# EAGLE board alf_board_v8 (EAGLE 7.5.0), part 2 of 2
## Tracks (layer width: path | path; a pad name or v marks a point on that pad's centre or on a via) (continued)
DB5  (via drill 0.61) (continued)
  Top 0.254: 73.12,115.5 R7.2 | IC7.19 65.12,68.5 66.62,70 66.62,78.62 68.62,80.62 68.62,112.38 70,113.75 72.75,113.75 73.24,114.24 R7.2 | v67.5,124.88 69.62,122.75 69.62,120.38 73,117 73,115.88 73.12,115.75 73.12,115.62 R7.2 | v183.25,56.88 196.25,56.88 198.5,54.62 IC12.32 | v176,61 v178,61 | v140.5,69 139,70.5 135.12,70.5 132.5,73.12 123.75,73.12 123.75,68.62 122.62,67.5 120.25,67.5 | 120.25,67.5 120.25,65.62 121.88,64 IC2.7 | v117,67.88 120.25,67.88 120.25,67.5
  Bottom 0.254: v67.5,124.88 43.38,124.88 41.75,126.5 CN1.37 | IC2.7 122,64 124.38,66.38 130.75,66.38 IC6.13 | v183.25,56.88 181.75,58.38 181.75,61 v178,61 | v176,61 170.38,66.62 142.88,66.62 v140.5,69 | v117,67.88 111.38,67.88 108.88,65.38 79,65.38 76,68.38 65.12,68.38 IC7.19
DB6  (via drill 0.61)
  Top 0.254: v129.62,47.12 127.75,49 v127.75,59.25 127.75,65.98 IC6.12 | v81.88,121 81.88,115.62 R6.2 82,115.5 82.88,114.62 82.88,101.88 84.25,100.5 84.25,87.62 83.5,86.88 v83.5,74.38 83.5,72.75 v82.5,71.75
  Bottom 0.254: v127.75,59.25 122.38,59.25 122,58.88 IC2.5 | v129.62,47.12 140.25,47.12 143.62,50.5 197.12,50.5 201.12,54.5 IC12.31 | v81.88,121 79.75,123.12 61.12,123.12 60.38,123.88 46.25,123.88 45.5,123.12 42.62,123.12 39.25,126.5 CN1.39 | v82.5,71.75 65.88,71.75 65.12,71 IC7.20 | v83.5,74.38 90.88,74.38 94,71.25 103,71.25 103.88,70.38 104,70.38 104,68.62 105.12,67.5 105.88,67.5 109,69 109,72.62 127.12,72.62 130.75,69 IC6.12
DB7  (via drill 0.61)
  Top 0.254: IC6.11 130.75,71.5 126.88,67.62 126.88,55.73 v126.15,55 | v176,64.25 179.57,60.62 179.57,53.62 187.25,46 187.25,42.38 194.38,42.38 203.7,51.7 IC12.30 | v90.5,114.12 90.5,115.5 R5.2 | 84.38,79.5 84.38,87 84.75,87.38 84.75,100.75 84.38,101.12 v84.38,114 | 84.38,79.5 v84.38,72.62 | CN1.41 36.62,126.5 36.62,121.62 41.05,117.2 v41.05,115.95 | v84.5,79.5 84.38,79.5
  Bottom 0.254: v176,64.25 173.12,67.12 144.88,67.12 139.38,72.62 131.88,72.62 130.88,71.62 IC6.11 130.75,71.62 128.38,74 110.38,74 104.88,79.5 v84.5,79.5 | IC4.13 95.38,110.12 97,111.75 97.75,111.75 97.75,113 96.75,114 90.62,114 v90.5,114.12 84.5,114.12 v84.38,114 84.25,114 83.62,114.62 42.38,114.62 v41.05,115.95 | v84.38,72.62 66,72.62 65.12,73.5 IC7.21 | v126.15,55 124.9,53.75 IC2.3
DR0  (via drill 0.61)
  Top 0.254: v58.5,33.75 58.5,43.25 R22.2 | IC11.3 90.5,10.25 90.5,13.12 89.5,14.12 v89.5,29.1 | v67.75,28.5 68.12,28.12 68.12,11.38 67.25,10.5 52.55,10.5 51,12.05 51,14 50.08,14.92 IC10.2
  Bottom 0.254: v58.5,33.75 65.12,33.75 69.06,29.81 | 69.06,29.81 69.38,29.5 89.1,29.5 v89.5,29.1 | 69.06,29.81 v67.75,28.5
DR1  (via drill 0.61)
  Top 0.254: 53.38,43.12 R21.2 53.46,40.46 53,40 50.3,40 47.45,37.15 47.45,34.95 45.62,33.12 45.62,19.12 47.25,17.5 IC10.3 48.55,16.25 63.75,16.25 65.88,14.12 v65.88,14 | v91.55,13.8 91.55,11.3 91.5,10.25 IC11.4
  Bottom 0.254: v65.88,14 66.62,14.75 90.6,14.75 v91.55,13.8
DR2  (via drill 0.61)
  Top 0.254: 38,21.62 38,31.25 42.3,31.25 42.3,39.05 43.25,40 47,40 48.43,41.43 R20.2 48.38,43.12 | 38,21.62 39.62,20 IC10.15 | v40.62,8.62 38,11.25 38,21.62 | IC11.6 93.59,7.84 v93.25,7.5
  Bottom 0.254: v93.25,7.5 92.5,8.25 41,8.25 v40.62,8.62
DR3  (via drill 0.61)
  Top 0.254: v37.12,17.5 37.12,32.25 41.12,36.25 41.12,40.88 43.38,43.12 R19.2 | IC11.7 94.62,10.12 94.6,8.25 94.6,7.45 v94.85,7.2
  Bottom 0.254: IC10.17 39.62,15 v37.12,17.5 37,17.5 34.12,20.38 27.62,20.38 27.62,19.12 37.25,9.5 42.38,9.5 43.12,8.75 93.5,8.75 v94.85,7.2
DR4  (via drill 0.61)
  Top 0.254: R18.2 107.12,43.25 106.88,43 106.88,36.88 107.62,36.12 107.62,20.75 105.62,18.75 99.12,18.75 IC11.14 99,18.62 95,18.62 v94.38,18
  Bottom 0.254: v94.38,18 74,18 73.5,18.5 60.25,18.5 60.25,16.62 61.88,15 IC9.2
DR5  (via drill 0.61)
  Top 0.254: v102.62,31.38 102.5,31.5 102.5,43.12 102.38,43.25 R17.2 | IC11.16 99,20.75 93,20.75 | v91.12,17.12 93,19 93,20.75 | v93.8,27.2 93,26.4 93,21 93,20.75
  Bottom 0.254: v91.12,17.12 90.75,17.5 62,17.5 IC9.3 | v102.62,31.38 102.38,31.38 98,27 94,27 v93.8,27.2
DR6  (via drill 0.61)
  Top 0.254: 55.44,24.06 55,23.62 52.62,23.62 52.62,21.75 54.25,20.12 IC9.15 | 55.44,24.06 56,24.62 56,29 56.5,29.5 56.5,32.12 58.12,32.12 62.12,36.12 62.12,42 63.38,43.25 R16.2 | v96.38,21.75 99,21.75 IC11.17 | v64,22.62 62.62,24 55.5,24 55.44,24.06
  Bottom 0.254: v64,22.62 93.5,22.62 94.38,21.75 v96.38,21.75
DR7  (via drill 0.61)
  Top 0.254: v97.25,29.88 97.25,43.25 R15.2 | IC11.20 99,24.75 95.28,24.75 | v95.28,28.02 95.28,24.75 | 95.28,24.75 v95.28,23.38 | v64.5,13.88 64.33,13.7 55.59,13.7 IC9.17
  Bottom 0.254: v64.5,13.88 65.88,15.25 91.25,15.25 92.65,16.65 97.65,16.65 98,17 98,23 97.62,23.38 v95.28,23.38 | v95.28,28.02 95.3,28 96,28 97.25,29.25 v97.25,29.88
G  (via drill 0.61)
  Top 0.254: IC11.12 99,16.62 96.72,16.62 96.4,16.3 96.4,12.6 99.12,9.88 122.12,9.88 123.5,11.25 JP3.3 123.5,11.38 123.12,11.75 123.12,28.88 114.38,37.62 v114.38,43.42 | 168.88,114.38 168.62,115.12 R44.2 | v98.5,56.62 96.38,58.75 96.38,91.88 v94.75,93.5
  Top 0.406: v168.88,112.75 168.88,114.38
  Bottom 0.254: v168.88,112.75 163.38,109.25 144.38,109.25 143.75,108.62 128.25,108.62 127.88,109 121.88,109 118.25,105.38 IC21.10 | v98.5,56.62 104.38,56.62 105,56 105,52.8 v114.38,43.42 | v94.75,93.5 95.62,94.38 113.38,94.38 115,96 115,100.15 116.4,101.55 119.95,101.55 120.5,102.1 120.5,104.55 119.7,105.35 IC21.10 | 118.25,105.25 IC21.10
GND  (via drill 0.6, 0.6 pad 0.25, 0.6 pad 2.18, 0.61)  (7 unrouted)
  Top 0.254: 134.38,109.25 134.12,109 C23.2 134,108.88 | 134.38,115.88 C22.- 134.5,116 | 143.5,90.38 R54.1 | 143.5,97.12 R55.1 143.5,97.25 | 144.88,115.25 R48.1 | 140.25,124.38 H5.B3,2 | 143.5,116.5 143.56,116.56 | 135.88,124.38 X2.2 | 134,106.75 133.82,106.62 | 125.88,105.38 IC21.7 | 156.88,90.25 R56.1 | 160.88,90.25 R57.1 160.88,90.38 | 155.88,109.12 R52.1 | 161.88,109.12 R51.1 161.75,109.12 | 161,115.12 R49.1 160.88,115.25 160.5,115.62 | 160.5,124.5 X3.1 | v44.75,23.12 45.12,23.5 45.12,29.5 44.88,29.75 44.88,31.25 44.05,32.08 C4.1 44.12,37 | IC18.8 189.5,19.38 190.25,18.62 190.25,15.62 190.29,15.5 | 19.25,19.88 C2.- | 15.25,20.5 S1.3 15.12,20.62 | 8.62,20.62 S1.4 8.75,20.62 | IC3.7 105.5,69.25 105.88,69.62 105.88,75 106.5,75.62 106.5,81.88 105.62,82.75 IC5.7 105.62,82.88 106.75,84 106.75,85.5 108.38,87.12 108.38,90.75 110.62,93 111,93 | IC16.3 183.25,59 180.75,59 IC16.2 180.75,59.12 180.5,59.38 180.5,64.12 178.25,66.38 IC16.14 | 188.38,66.62 IC16.10 | 204.38,29.75 IC17.13 | 105.62,102.38 IC4.8 | 148.93,15.5 148.88,15.62 147.88,16.62 147.88,29.62 146.25,31.25 IC13.8 | IC18.13 179.25,27.12 178.38,28 178.38,28.62 178,29 178,36.75 178.3,37 | 86.62,10 86.62,10.12 | 109.88,124.38 X1.2@1 | IC11.63 86.62,10.25 86.6,12.47 86.6,22.6 88,24 88,29 88.59,29.59 IC11.32 88.62,32.12 | v51.5,81 51.5,70.5 50.7,69.7 48.9,69.7 48.25,69.05 48.25,64.85 49.75,63.35 IC7.16
  Top 0.406: 228.8,138.95 229,139 | 178.25,72 178.15,71.9 | 178.15,66.58 IC16.14 | R28.1 | 229,72.35 229.35,72 229.15,71.8 229.15,58.85 229.11,58.89 | R66.2 C30.- | C30.- 191.95,113.95 190,113.95 | 190,113.95 C29.2 | IC22.24 190,107.63 190,113.95 | C35.- 211.4,123.05 C34.2 211.3,117.85 R71.1 v213,110 C38.1 | C30.- v192,116 | 229,104.18 229,104 | 229,99.1 229,99 | 214.45,99.8 C37.1 | 229,109.05 229,109 | IC19.10 226.12,23 | 182.46,72 183,72 | 191.46,72 191,72 | 200.46,72 200,72 | 209.46,72 209,72 | C42.2 155,16.05 C43.- 148.93,15.5 X4.1 | C40.2 197,16.05 C41.- 190.29,15.5 X5.1 | 143.5,97.12 143.5,90.38 | 144.88,115.25 143.56,116.56 143.56,120.44 143,121 140.69,121 X2.2 | 125.88,105.38 132.43,105.38 133.82,106.62 | 134,108.88 134,106.75 | 204.38,37 204.38,29.75 | v86.62,3.88 86.62,10 86.62,10.25 | 160.5,124.62 X3.1 | v25.45,74 v25.45,71.12 | 160.88,96.12 160.88,96.25 | 156,107 155.84,107.16 | 143.5,97.25 142.85,97.9 142.85,113.15 144.89,115.19 R48.1 | 204.4,135.15 X7.SH2 | 210.8,134.75 X7.SH1 | 197.65,138.6 arc-90 198,138.95
  Top 0.813: 178.15,71.9 178.15,66.58 | R36.1 159,81.23 | 159,81.23 R28.1 | 229.11,58.89 IC14.7 | IC22.24 190.03,102.5 | 190.03,102.5 IC22.1 | 190.03,102.5 197.65,102.5 IC22.7 197.65,97.3 C36.2 198.3,95.35 198.9,94.75 C27.2 205.25,93.5 C28.- 211.75,93.5 214.45,96.2 v214.45,97.85 214.45,99.8 | IC23.13 229,104.18 | IC23.11 229,99.1 | 226.12,23 229.31,23 | R61.A 182.46,72 | R62.A 191.46,72 | R63.A 200.46,72 | R60.A 209.46,72 | CN1.48 29.16,138.95 29,138.95 | CN1.2 86.66,138.95 87,138.95 | 121.99,77 111,77 111,93 111,102.38 | 111,102.38 111,121 109.88,121 | 109.88,121 105,121 105,138.95 | IC2.10 121.99,77 | 121.99,77 138.4,77 IC6.10 | IC12.1 178.3,37 204.38,37 229.32,37 | 134.38,115.88 134.38,109.25 | 134.5,116 135.88,117.38 135.88,124.38 | 160.88,90.25 159,90.25 | 159,90.25 156.88,90.25 | 160.88,90.38 160.88,96.12 | 159,90.25 159,81.23 | 158.88,107 161.88,107 161.88,109.12 | 158.88,107 156,107 | 161,115.12 161,110.72 161.75,109.12 | 160.5,115.62 160.5,124.5 | 160.88,96.25 158.88,97.25 158.88,107 | 19.25,19.88 15.25,19.88 15.25,20.5 | 8.62,20.62 8.25,21 8.25,26.12 IC1.7 | 8.75,20.62 15.12,20.62 | 188.38,72 188.38,66.62 | 111,102.38 105.62,102.38 | 161,138.95 161,124.62 160.5,124.62 | 109.88,121 109.88,124.38 | 155.84,107.16 R52.1
  Top 1.27: 210.8,134.75 X7.5 204.4,135.15 X7.3 198,134.75 X7.SH3 197.65,138.6
  Top 1.422: 229.35,72 229.32,37 229.31,23 229.3,5 H3.B3,3
  Top 2.184: 9.7,135 9.75,138.95 29,138.95 87,138.95 105,138.95 161,138.95 198,138.95 228.8,138.95 | 229.35,72 209,72 200,72 191,72 188.38,72 183,72 178.25,72 | H1.B3,3 9.7,135 | 229,72.35 229,99 229,104 229,109 229,135 | 229,135 229,139 | H2.B3,3 229,135 | X1.2@1 X1.2@2 X1.2 X2.2@1 X2.2@2 X2.2 142.5,125.39 H5.B3,2 | X6.2 X6.2@2 X6.2@1 167.5,125.46 H6.B3,2 | v9.7,105.55 arc90 9.75,105.6 C47.- 11,111 11,119.39 J1.TIP 9.7,121.91 9.7,135
  Bottom 0.254: 29.62,71.12 IC8.29 29.5,71.12 | 49.75,63.38 IC7.16 | v51.5,81 64.88,81 65,81.12 IC7.24 | IC21.4 125.75,97.75 123.62,99.88 122.12,99.88 C14.1 | 125.75,105.38 IC21.7 | IC9.1 61.88,12.5 59.38,15 58.12,15 58,15.07 | v44.75,23.12 43.75,22.12 43.12,22.12 C13.1 | 40.79,13.12 40.88,13 46.75,13 47.25,12.5 IC10.1 47.38,12.5 | 54.25,12.5 IC9.18 | IC18.13 179.38,27 183.25,23.12 183.25,22.97 | IC17.13 204.5,29.62 208,26.12 208,25.97 | C16.1 134.88,61.88 133.88,61.88 133.88,52.88 132.22,51.22 IC6.19 | IC12.24 219,54.62 220.5,56.12 220.5,62.5 220.62,62.5 C10.1 | C11.1 168.62,38.12 177.12,38.12 178.25,39.25 IC12.1 | 149.99,34.12 150.12,34 151.75,32.38 165.75,32.38 165.84,32.25 | 8,26.38 IC1.7
  Bottom 0.406: C19.1 12,29.1 IC1.7 | IC10.18 40.79,13.12 43,14.66 C13.1 42.25,21.3 37.65,21.3 36.95,22 16,22 15.22,21.22 S1.3 | C20.1 58,15.07 IC9.18 | C12.1 118,68.54 IC2.10 | C16.1 135,69.15 IC6.10 | C18.1 103.24,72.45 IC3.7 | C21.1 103.26,86.1 IC5.7 | C17.1 103.35,105.55 IC4.8 | C14.1 122,104.08 124.52,106.6 | 124.52,106.6 IC21.8 | C9.1 149.99,34.12 IC13.8 | C46.1 183.25,22.97 186.97,22.97 IC18.8 | C45.1 208,25.97 211.66,25.97 IC17.8 | C44.1 225.06,24.06 IC19.10 | C10.1 224.07,62.49 IC14.7 | C5.1 187.4,65.63 IC16.10 | C11.1 168.49,34.17 165.84,32.25 IC20.7 | C15.1 221.45,94.29 IC23.7 | v192,116 191.59,116 X6.2 | IC23.11 C15.1 | C15.1 219.85,97.85 v214.45,97.85 arc-90 213,99.3 v213,110 | 29.62,71.12 32.52,69.72 43.3,69.72 49.75,63.38 | 124.52,106.6 125.75,105.38 | 47.38,12.5 54.25,12.5 | v86.62,3.88 86.62,1 | 1,69.88 16.45,69.9 17.48,71.12 v25.45,71.12 29.5,71.12 | C3.1 v25.45,74 | JP4.2 19.3,11.38 | 1.45,67.65 1.45,66.45 arc-90 1,66
  Bottom 0.813: JP3.2 126,8.73 126,1 | 1,26.38 8,26.38 | 19.3,11.38 19.3,1.79
  Bottom 1.016: 1.45,67.65 1,67.65
  Bottom 2.184: 126,1 86.62,1 19.3,1.79 1,2 1,5 | 1,5 1,26.38 1,66 1,67.65 1,69.88 1,103 arc-90 3.55,105.55 v9.7,105.55 | 1,5 H4.B3,3
  other vias: 176,131 194,135 224,122.3 180,102 176,91 224,112 180,114
  pour Bottom (isolate 0.813): 173,140 230,140 230,109 213,109 213,86 173,86
  pour Top (isolate 1.016): 173,140 230,140 230,109 213,109 213,86 173,86
  pour Bottom (isolate 0.813): 230,0 0,0 0,15 37,15 37,6 230,6
  pour Top (isolate 0.254): 0,140 13,140 13,125 0,125
  pour Top (isolate 0.813): 230,0 207,0 207,3 207,12 230,12
KD0  (via drill 0.61)
  Top 0.254: v207.12,7.75 210.62,11.25 210.62,20.88 209.5,22 IC17.6 | IC11.1 88.62,10.12 88.62,5.7 v93.15,5.7 | v123.88,5.88 127.78,5.88 v127.8,5.85
  Bottom 0.254: v207.12,7.75 129.7,7.75 v127.8,5.85 | v93.15,5.7 123.7,5.7 v123.88,5.88
KD1  (via drill 0.61)
  Top 0.254: v174.62,6.88 175.88,6.88 179,10 179,13 181.38,15.38 v182.88,15.38 | v123.97,3.92 v127.83,3.92 | IC11.2 89.59,7.16 v90.03,6.72
  Bottom 0.254: v182.88,15.38 192.62,15.38 199.25,22 IC17.2 | v90.03,6.72 92.83,3.92 v123.97,3.92 | v127.83,3.92 130.78,6.88 v174.62,6.88
KD2  (via drill 0.61)
  Top 0.254: v138.12,9.5 138.12,4.88 206.25,4.88 213.25,11.88 213.25,31.75 212.75,32.25 v211.62,32.25 | v93.88,15 92.62,15 92.62,10.25 IC11.5
  Bottom 0.254: v211.62,32.25 201.88,32.25 199.38,29.75 IC17.15 | v138.12,9.5 133,14.62 108.5,14.62 108.12,15 v93.88,15
KD3  (via drill 0.61)
  Top 0.254: IC11.8 95.62,10.25 95.62,9.9 v96.83,9.9
  Bottom 0.254: IC17.3 194.25,14.5 148.88,14.5 143,8.62 127.75,8.62 126.5,9.88 96.83,9.88 v96.83,9.9
KD4  (via drill 0.61)
  Top 0.254: IC11.9 99.12,13.62 99,13.5 99,12 99.35,11.65 102.85,11.65 104.5,13.3 v104.5,17.43
  Bottom 0.254: v104.5,17.43 104.5,20.88 105.38,21.75 173.38,21.75 173.57,22.15 176.57,22.15 176.75,21.88 186.62,21.88 188,20.5 arc-45 188.25,19.9 188.25,17.95 188.9,17.3 189.9,17.3 191.1,18.5 193.25,18.5 196.75,22 IC17.1
KD6  (via drill 0.61)
  Top 0.254: v138.12,19.5 144.75,12.88 144.75,5.38 206,5.38 212,11.38 IC17.7 | v105.38,20.5 102.25,23.62 99.12,23.62 IC11.19
  Bottom 0.254: v138.12,19.5 137.62,20 105.88,20 v105.38,20.5
KJ0  (via drill 0.61)
  Top 0.254: v134.88,29.62 v134.88,43.5
  Bottom 0.254: v134.88,43.5 133.88,44.5 126.75,44.5 126.75,46.38 122,51.12 IC2.2 | v134.88,29.62 135.12,29.88 163.38,29.88 163.5,30 171.38,30 174.25,27.12 IC18.15
KJ1  (via drill 0.61)
  Top 0.254: v123.75,46.12 123.75,54.5 122,56.25 IC2.4 | v169.25,28.12 169.25,21.88 171.62,19.5 IC18.1 | v134,28.75 134,43.12 v133.5,43.62
  Bottom 0.254: v123.75,46.12 126.25,43.62 v133.5,43.62 | v134,28.75 137.38,28.75 138,29.38 163.62,29.38 163.75,29.5 167.88,29.5 v169.25,28.12
KJ2  (via drill 0.61)
  Top 0.254: v120.25,46.12 120.25,59.62 121.88,61.25 IC2.6 | v120.25,42.38 124.12,38.5 124.12,32.62 v135.88,20.88
  Bottom 0.254: v120.25,42.38 v120.25,46.12 | v135.88,20.88 136.12,21.12 172.62,21.12 174.25,19.5 IC18.2
KJ3  (via drill 0.61)
  Top 0.254: v124.62,47.25 124.62,63.75 122,66.38 IC2.8 | v135.88,19.12 123.62,31.38 123.62,36.12 118.75,41 118.75,43.25 119.38,43.88 v121.12,43.88
  Bottom 0.254: v124.62,47.25 124.38,47 123.38,47 121.12,44.75 v121.12,43.88 | v135.88,19.12 137.25,17.75 175.12,17.75 176.75,19.38 IC18.3
KJ4  (via drill 0.61)
  Top 0.254: v118,75.88 118,75.25 114.38,71.62 IC2.11 | v146.88,68.88 147.75,68 v147.75,65.5 | v152.5,60.75 157.62,55.62 157.62,25.77 160.4,23 164.2,23 165.1,23.9 167.8,23.9 168.25,23.45 168.25,20.75 v172.62,16.38
  Bottom 0.254: v118,75.88 118.38,76.25 139.5,76.25 v146.88,68.88 | v152.5,60.75 v147.75,65.5 | v172.62,16.38 173,16.75 181.75,16.75 184.38,19.38 IC18.6
KJ5  (via drill 0.6 pad 0.41)
  Top 0.406: v217,89 v217,86 | v209,88 v200,88 | v112.2,75.45 111.3,74.55 v111.3,71.75 | v112,69 111.75,68.75 v111.75,66.4
  Bottom 0.406: IC23.8 225.26,89 v217,89 | v217,86 214,86 212,88 v209,88 | v112.2,75.45 112.2,78.2 119,85 133,85 136,88 v200,88 | v111.3,71.75 112,71.05 v112,69 | v111.75,66.4 111.8,66.45 IC2.13
KJ6  (via drill 0.61)
  Top 0.254: IC2.15 112.62,59.62 112.62,36.62 122.25,27 v122.25,19.12
  Bottom 0.254: v122.25,19.12 124.12,17.25 177.12,17.25 179.25,19.38 IC18.4
KJ7  (via drill 0.61)
  Top 0.254: v110.88,59.75 110.88,70.12 v116.62,75.88 | v214.75,81.38 215,81.62 215,92 217.02,94.02 IC23.6
  Bottom 0.254: v110.88,59.75 114.25,56.38 IC2.17 | v116.62,75.88 118.12,77.38 181.12,77.38 182,76.5 209.88,76.5 v214.75,81.38
N$1
  Top 0.406: R65.1 199.1,92 212,92 215.55,95.55 215.55,97.7 216.95,99.1 IC23.4
N$2
  Bottom 0.254: C1.1 28.12,37.62 29.5,39 29.5,41.88 28.12,41.88 R1.2 | IC1.2 8.12,39 5.88,40.65 5.88,42.9 6.97,44 19,44 21.1,41.9 R1.2 | 28,42 R1.2
N$3  (via drill 0.61)
  Top 0.254: v13.62,36.38 8.25,36.38 IC1.3
  Bottom 0.254: v13.62,36.38 14.62,35.38 18.38,35.38 20,37 22,37 23.37,35.63 C1.2 | 27.75,36 28,35.75 C1.2 | C1.2 29.63,35.63 30,36 30,37 30.53,37.53 R2.1
N$4
  Bottom 0.254: R1.1 28,40 27.75,39.75 21.12,39.75 Q1.1 21,39.75 18.25,42.5 9.25,42.5 8.25,41.5 IC1.1
N$5  (via drill 0.6, 0.61)
  Top 0.254: v177.12,36.38 177.12,29.12 177.88,28.38 177.88,26.38 178.38,25.88 178.38,23 181.88,19.5 IC18.5 | v190,43.25 199.62,52.88 199.62,55.75 192.62,62.75 v181.38,62.75 | v178.12,64.5 176.5,66.12 176.5,74.5 177.1,75.1 v177.3,75.1 | v207.75,75.1 207.75,84.75 211,88 211,90 217.56,96.56 IC23.5
  Bottom 0.254: v181.38,62.75 179.62,64.5 v178.12,64.5 | v177.12,36.38 188.38,36.38 189.7,37.7 189.7,42.95 v190,43.25 | v207.75,75.1 v177.3,75.1
N$6  (via drill 0.61)
  Top 0.254: v175.55,21.12 170.75,21.12 170.75,25.25 v170.12,25.88 | v164.12,28.62 163.12,29.62 163.12,49 165.12,51 165.12,64.75 v170.25,69.88
  Top 0.406: v214.5,76 220,76 222,78 222,93 223.02,94.02 IC23.9
  Bottom 0.254: v175.55,21.12 185.25,21.12 186.88,19.5 IC18.7 | v170.12,25.88 167.38,28.62 v164.12,28.62 | v170.25,69.88 176.38,76 v214.5,76
N$7  (via drill 0.61)
  Top 0.254: v102.5,55.25 104.5,57.25 104.5,75.75 105.5,76.75 IC3.8 | v20.82,52.15 20.82,44.83 18,42 18,40 16.94,38.94 IC1.13
  Bottom 0.254: v102.5,55.25 99.38,52.12 20.85,52.12 v20.82,52.15
N$8
  Top 0.254: 22.62,16.88 R3.1 | 19.38,16.88 C2.+ 19.25,16.75 | 15.25,16.12 S1.1 15.12,16.12 | 8.12,31.25 IC1.5 | 8.62,16.12 S1.2 8.75,16.12
  Top 0.406: JP4.1
  Top 0.813: 19.38,16.88 22.62,16.88 | 19.25,16.75 15.25,16.75 15.25,16.12 | 8.12,31.25 4.38,29.5 4.38,18.38 8.62,16.12 | 8.75,16.12 15.12,16.12 | JP4.1 C2.+
N$9
  Bottom 0.254: IC4.7 102.88,102.38 98.25,97.75 81.25,97.75 JP1.1
N$10  (via drill 0.61)
  Top 0.254: v101.25,55.75 101.5,56 101.5,75.75 100.5,76.75 IC3.10 | v35.4,38.75 35.4,41.4 36.35,42.35 v36.35,53
  Bottom 0.254: v36.35,53 98.5,53 v101.25,55.75 | IC1.10 15.88,31.25 16.75,30.38 33.38,30.38 34.65,31.65 34.65,38 v35.4,38.75 | IC3.12 95.38,76.75 97,75.12 98.75,75.12 100.38,76.75 IC3.10
N$11  (via drill 0.61)
  Top 0.254: v96.88,107 96.88,70.25 97.88,69.25 IC3.4
  Bottom 0.254: v96.88,107 95.62,108.25 94.62,108.25 92.88,110 IC4.14
N$12  (via drill 0.61)
  Top 0.254: v108.5,73.62 109,73.12 109,57 v108.62,56.62
  Bottom 0.254: IC2.1 121.88,48.62 120.88,47.62 112.62,47.62 112.62,49.5 114.25,51.12 IC2.19 114.12,51.12 v108.62,56.62 | v108.5,73.62 104.5,73.62 104.5,77.38 103.38,78.5 99.62,78.5 98,76.88 IC3.11
N$13
  Top 0.254: IC3.1 90.25,69.25 89.25,70.25 89.25,109 90.25,110 IC4.15
N$14
  Top 0.254: IC19.11 226,25.62 221,30.62 218.5,30.62 IC19.2 | IC18.12 182,27.12 183.62,28.75 185.88,28.75 185.88,24.62 188.25,22.25 188.25,13.25 190,11.5 199.88,11.5 199.88,10.38 X5.12
  Bottom 0.254: IC17.12 207,29.75 208.62,31.38 217.75,31.38 218.38,30.75 IC19.2 | 198.81,9.19 199.88,10.25 X5.12 | 198.81,9.19 198.25,8.62 160.25,8.62 158.62,10.25 X4.12 | IC19.11 226.12,25.5 227.75,23.88 227.75,14.5 213.88,14.5 208.5,9.12 198.88,9.12 198.81,9.19
N$15  (via drill 0.61)
  Top 0.254: v83.75,42.38 83.75,61.88 83.88,62 R25.2 | IC11.21 99,25.75 97.12,25.75 96.38,26.5 v96.38,40.75
  Bottom 0.254: v83.75,42.38 85.38,40.75 v96.38,40.75
N$16
  Top 0.254: 208.75,54.62 IC12.28
  Top 0.813: R38.2 204.75,60.5 208.75,56.25 208.75,54.62
  Bottom 0.254: IC12.25 216.38,54.62 214.75,56.25 210.5,56.25 208.88,54.62 IC12.28
N$17  (via drill 0.61)  (1 unrouted)
  Top 0.254: 146.88,115.25 R48.2 146.88,115.12 | 146.88,109.25 R43.1 146.88,109.12
  Top 0.406: 146.88,115.25 146.88,119.62 D1.A | 146.88,115.12 146.88,109.25 | v147.38,107 146.88,107.5 146.88,109.12
  Bottom 0.406: 168.62,103.25 167.47,104.4 156.72,104.4 154.28,106.85 147.53,106.85 v147.38,107
N$18
  Top 0.254: 139.25,115.88 139.88,115.25 R47.2 | 139.25,119.62 D1.C
  Top 0.406: 139.25,119.62 139.25,115.88
N$19  (via drill 0.61)
  Top 0.254: 162.75,115.25 R49.2
  Top 0.406: 162.75,115.25 162.72,115.28 v162.72,120.95 | v171.5,81 171,81.5 171,105 170.38,105.62 168.75,105.62 168.69,105.69 T1.E
  Bottom 0.254: R61.E 185,81 v171.5,81
  Bottom 0.406: X3.2 157.77,124.23 161.05,120.95 v162.72,120.95 163.1,120.95 163.6,120.45 170.6,120.45 170.6,106.3 169.99,105.69 T1.E
N$20  (via drill 0.6 pad 0.25)
  other vias: 195.1,112.45
N$21  (via drill 0.61)
  Top 0.254: 166.38,115.62 166.75,115.25 R44.1 | 163.75,109.25 R51.2
  Top 0.406: v166.38,116.75 166.38,115.62 | v163.75,113.12 163.75,109.25 | T2.B 161.75,103 164,103 165,104 165,109 164.76,109.24 R51.2
  Bottom 0.406: v166.38,116.75 165.38,115.75 163.75,115.75 | 163.75,115.75 152.65,115.75 D2.A | 163.75,115.75 v163.75,113.12
N$22  (via drill 0.61)
  Top 0.254: 140,109.12 R50.2
  Top 0.406: 140,109.12 140.5,108.62 v140.5,107.62
  Bottom 0.254: v140.5,107.62 140.88,108 152.52,108 D2.C
N$23  (via drill 0.61)
  Top 0.254: 157.62,109.25 R52.2 157.75,109.12 | 155,124.5 X3.3
  Top 0.406: 157.62,109.25 157.62,121.85 156.88,122.62 155,124.5 | v159.9,108.28 158.94,109.24 R52.2 | v169.38,107.12 170.88,107.12 172,106 172,83 173,82 196.54,82 R62.E
  Bottom 0.406: v169.38,107.12 169.1,107.4 161.65,107.4 161.63,107.38 | 161.63,107.38 T2.E | v159.9,108.28 160.79,107.38 161.63,107.38
N$24  (via drill 0.6 pad 0.25)
  Top 0.406: IC22.17 198.92,105.45 v198.9,105.45 | v188.15,105.1 186.05,105.1 arc90 R67.2
  Bottom 0.406: v198.9,105.45 arc-90 198.55,105.1 v188.15,105.1
N$25
  Top 0.254: IC12.27 211.38,54.62 212.88,56.12 212.88,67.5 213.62,68.25 219,68.25 219,66.62 IC14.11
N$26  (via drill 0.61)
  Top 0.254: IC5.4 98,82.75 99.38,81.38 99.38,56.38 102.62,53.12 102.62,46.17 103.8,45 103.8,41.3 104.75,40.35 104.75,37.45 106.08,36.12 v106.08,35.88 | v171.75,25 172.75,26 172.75,27.62 176,30.88 176,39.12 177.5,40.62 177.5,43.62 186.25,43.62 186.75,43.12 186.75,41 210,41 222.62,53.62 222.62,65 IC14.9 | v147,26.38 144,29.38 144,33 144.88,33.88 146.12,33.88 IC13.7
  Bottom 0.254: v106.08,35.88 144.25,35.88 146.12,34 IC13.7 | v171.75,25 150.5,25 149.12,26.38 v147,26.38
N$27  (via drill 0.61)
  Top 0.254: v210.12,48.75 215,53.62 215,65.5 214,66.5 IC14.13 | v166.75,37.83 166.75,37.88 v169.88,41
  Bottom 0.254: v169.88,41 170.25,40.62 174.62,40.62 176.25,42.25 185.12,42.25 185.5,41.88 187.38,41.88 194.25,48.75 v210.12,48.75 | v166.75,37.83 162.95,37.83 161.57,36.45 IC13.11
N$28  (via drill 0.61)
  Top 0.254: v103,87.12 103,85.38 100.5,82.88 IC5.5 | v150,60.75 152.12,58.62 152.12,35.62 153.75,34 IC13.10
  Top 0.406: v144,65 143,66 143,80 135.12,87.88 v130.25,87.88
  Bottom 0.254: v144,65 148.25,60.75 v150,60.75
  Bottom 0.406: v130.25,87.88 110.88,87.88 110,87 108,87 107,88 104.85,88 104.1,87.25 103.12,87.25 v103,87.12
N$29  (via drill 0.61)
  Top 0.254: v205.88,41.88 217.62,53.62 217.62,62.75 | 217.62,62.75 217.62,65.5 216.62,66.5 IC14.12 | IC14.10 221.5,66.5 217.75,62.75 217.62,62.75
  Bottom 0.254: v205.88,41.88 192.5,41.88 192.5,38.75 189.25,35.5 171.75,35.5 166.75,30.5 154.62,30.5 153.88,31.25 IC13.9
N$30  (via drill 0.61)
  Top 0.254: IC18.10 187,27.12 187,28 191,32 R41.1 191.12,32.12 194.38,35.38 v198,35.38 | v206.38,35.38 212,29.75 IC17.10
  Bottom 0.254: v198,35.38 v206.38,35.38
N$31
  Top 0.254: IC12.29 206.25,54.5 207.88,52.88 210.05,52.88 210.05,68.75 226.62,68.75 226.62,66.62 IC14.8
N$32
  Top 0.406: 154,74.86 R33.2 R34.1 150.64,70.81 R37.1 150.56,70.81 R35.1 | 154,74.86 150.41,74.86 C8.+ | R36.2 154,80.22 154,74.86
N$33
  Top 0.406: 164,74.86 R31.2 R32.1 167.31,70.81 R29.1 R30.1 | 164,74.86 167.54,74.86 C7.+ | R28.2 164,80.16 164,74.86
N$34  (via drill 0.6)
  Top 0.254: 138.12,103.12 R45.1 | 139.38,90.38 D3.A
  Top 0.406: R54.2 145,89.95 145,88 140,88 139.43,88.57 D3.A 138.74,90.26 137,92 137,102 138.12,103.12 138.12,100 v141,100
  Bottom 0.406: v141,100 144.16,103.16 T3.B
N$35  (via drill 0.61)
  Top 0.254: 186.19,14.56 190.38,10.38 191.62,10.38 X5.9 | 186.19,14.56 185.88,14.88 185.88,21.12 185.38,21.62 185.38,26.12 184.5,27 IC18.11 | v175.12,34.62 175.12,39 172.5,41.62 IC20.12 | X4.9 150.38,10.25 154.62,6 186.12,6 186.12,14.5 186.19,14.56 | IC17.11 208.12,28.38 v208.12,19.75
  Bottom 0.254: IC17.11 209.5,29.62 211.12,28 216.25,28 217.88,29.62 222.5,29.62 226,33.12 IC19.14 | v175.12,34.62 181,28.75 182.75,28.75 184.38,27.12 IC18.11 | X5.9 191.75,10.38 192.88,11.5 202.38,11.5 202.65,11.78 202.65,14.28 v208.12,19.75
N$36  (via drill 0.6)
  Top 0.254: v161,34 160,33 160,26 160.95,25.05 R39.1 162,25 166,25 C39.1
  Bottom 0.254: IC20.5 163.6,36.6 v161,34
N$37  (via drill 0.6, 0.61)
  Top 0.254: v176.88,52.38 177.05,53.1 177.05,58.35 178.12,58.88 IC16.1 | v161.9,39.15 161.9,36.86 R26.2 | Q2.2 171.25,57 168.25,57 168.25,41.25 166.14,39.14 IC20.4
  Bottom 0.254: v176.88,52.38 171.38,52.38 Q2.2 | IC20.4 v161.9,39.15
N$38  (via drill 0.61)
  Top 0.254: v161.5,48.12 161.5,48.38 160,48.38 R27.1 | Q2.1 166.38,52.38 165.62,51.62 165.62,47.62 164.88,46.88 IC20.1
  Bottom 0.254: v161.5,48.12 162.75,46.88 164.75,46.88 IC20.1
N$39  (via drill 0.6)
  Top 0.254: C6.1 159.99,45 | 159.99,45 159.99,46.56 R27.2 | v162,45 159.99,45
  Bottom 0.254: IC20.2 162.78,44.22 v162,45
N$40  (via drill 0.6)
  Top 0.254: v161.95,41.7 arc0 C6.2 159.99,38.76 R26.1
  Bottom 0.254: IC20.3 v161.95,41.7
N$41  (via drill 0.6)
  Top 0.406: R53.2 134.71,96.71 v135,97
  Bottom 0.406: v135,97 135.88,97.88 D3.C
N$42  (via drill 0.61)
  Top 0.254: 145.38,97.25 R55.2 145.38,97.12 | 145.38,100.5 T3.E
  Top 0.406: 145.38,100.5 145.38,97.25 | v149.25,86.12 149.25,93.33 R55.2 | v150.38,103.88 150.38,122.72 X3.4
  Bottom 0.254: R63.E 202.12,81.88 179.5,81.88 177.38,84 166,84 163.88,86.12 v149.25,86.12 | T3.E
  Bottom 0.406: v150.38,103.88 146.12,100.62 T3.E
N$43  (via drill 0.6, 0.61)
  Top 0.254: 162.75,90.25 R57.2 | X3.5 149.5,124.5 149.5,102.5 151.4,100.6 T4.E
  Top 0.406: 162.75,90.25 v162.75,92.75 163,93 169,93 169.45,92.55 169.45,80 179,80 180,79 v180,74
  Bottom 0.254: 152.38,100.5 T4.E
  Bottom 0.406: v162.75,92.75 153,100.5 152.38,100.5 | R60.E 217,76 217,74 v180,74
N$44  (via drill 0.61)
  Top 0.254: 132.12,109 C23.1 132.25,108.88 132.05,108.38 | 128.88,112.25 L1.2 128.88,112.38 | 131.38,115.88 C22.+
  Top 0.406: v132.05,107.2 132.05,108.38
  Top 0.813: 131.38,115.88 128.88,113.38 128.88,112.38 | 128.88,112.25 128.88,111.12 131.06,108.94 C23.1
  Bottom 0.254: 161.75,100.62 T2.C 161.62,100.62 | 168.62,100.62 T1.C | 145.38,105.75 T3.C 145.25,105.75 | 152.25,105.75 T4.C 152.38,105.62
  Bottom 0.406: 168.62,100.62 161.75,100.62 | 152.25,105.75 145.38,105.75 | v132.05,107.2 134.75,105.75 145.25,105.75 | 152.38,105.62 153.38,105.62 158.42,100.58 T2.C
N$45  (via drill 0.6)
  Top 0.406: X3.9 148.58,127.42 v144,132
  Bottom 0.813: R58.1 142.41,132 v144,132
N$46
  Top 0.254: R40.2 201,34 201.75,33.25 201.75,29.75 IC17.14 201.84,27.56 205.65,23.75 205.65,20.15 207.1,18.7 209.49,18.7 X5.8
N$47
  Top 0.254: IC19.9 226,20.62 218.5,28.12 IC19.3
N$48  (via drill 0.61)
  Top 0.254: v179,29.25 179,34 R42.1 | X4.8 168.25,12.88 172.38,12.88 177.88,18.38 177.88,25.62 176.88,26.62 176.88,27 IC18.14
  Bottom 0.254: v179,29.25 176.88,27.12 IC18.14
N$49
  Top 0.254: IC19.12 226,28.25 224.12,28.25 219.25,33.12 218.5,33.12 IC19.1
N$50
  Top 0.254: IC20.11 172.5,39.12 174.12,37.5 174.12,33.25 172.5,31.62 IC20.8 172.38,31.5 169.5,31.5 167.9,29.9 C39.2
N$51
  Top 0.254: 170.75,36.5 172.38,36.5 IC20.10 | 170.75,36.5 168.12,36.5 166.5,34.88 166.5,29.5 163.95,26.95 R39.2 | 170.75,36.5 170.75,42.5 172.38,44.12 IC20.13
N$52
  Top 0.406: C26.1 R61.S
N$53  (via drill 0.61)
  Top 0.254: v167.38,34.5 172.38,34.5 172.38,34.12 IC20.9
  Bottom 0.254: v167.38,34.5 165.25,34.5 164.88,34.12 IC20.6
N$54
  Top 0.406: C25.1 R62.S
N$55
  Top 0.406: C24.1 193.85,92.15 202.46,83.54 R63.S
N$56
  Top 0.406: IC22.3 192.57,98.57 191.65,97.65 C25.2
N$57
  Top 0.406: IC22.2 191.3,99.1 C26.2
N$58
  Top 0.406: IC22.4 C24.2
N$59
  Top 0.406: 214.88,106.72 arc-90 C38.2
  Top 0.813: IC23.1 214.88,106.72 | C38.2 210.44,107.15 arc90 Q3.1
  Bottom 0.406: R64.2 IC23.1
N$60
  Top 0.406: 217.64,101.75 IC23.3
  Top 0.813: 217.64,101.75 C37.2 210.84,101.75 arc-90 Q3.2 | IC23.3 IC23.2
  Bottom 0.406: R64.1 IC23.2
N$61  (via drill 0.6 pad 0.41)
  Top 0.406: IC22.10 201.46,98.54 202.1,97.9 v202.1,96.4
  Bottom 0.406: v202.1,96.4 202.1,93.44 R60.S
N$62  (via drill 0.6, 0.61)
  Top 0.254: 138,109.25 R50.1 137.88,109.12 | 138,115.12 R47.1 | 134.62,92.5 R53.1 | v109.25,88.75 109.25,74.88 109.88,74.25 109.88,73.62 109.5,73.25 109.5,52.62 109.12,52.25 109.12,18.12 115.88,11.38 JP3.9
  Top 0.406: 138,115.12 138,109.25 | 134.62,92.5 131.5,92.5 130,94 | 130,94 130,99 | 130,99 128.73,100.27 IC21.5 | 137.88,109.12 136,107.25 136,105 130,99 | v129,90 130,91 130,94
  Bottom 0.406: v129,90 127.75,88.75 v109.25,88.75
N$63
  Top 0.406: IC22.6 196.38,92.8 R65.2
N$64  (via drill 0.6 pad 0.25)
  Top 0.406: IC22.20 v195.11,112.44 v195.1,112.45 | v195.1,115.45 195.15,115.45 R68.2
  Bottom 0.406: v195.1,112.45 v195.1,115.45
N$65
  Top 0.406: IC22.9 C36.1
N$66
  Top 0.406: IC22.18 R66.1
N$67
  Top 0.406: IC22.16 R69.2
N$68
  Top 0.406: IC22.15 201.46,112.46 R70.2
N$69
  Top 0.813: R68.1 C33.+
N$70
  Top 0.406: 204.7,122.7 C32.+
  Top 0.813: R69.1 202.6,120.6 204.7,122.7
N$71  (via drill 0.6 pad 0.25)
  Top 0.406: R70.1 v204.75,115.9 | v214.9,115.9 218,115.9 C31.+
  Bottom 0.406: v204.75,115.9 v214.9,115.9
N$72
  Top 0.406: IC22.14 202.73,110.73 207,115 207,121.4 C35.+
N$73
  Top 0.406: C34.1 209.5,114.15 R71.2 209.35,114 209,114 204,109 IC22.13
N$74  (via drill 0.6 pad 0.25)
  other vias: 195.1,115.45
N$75
  Top 0.813: C33.- X6.1
N$76  (via drill 0.61)
  Top 0.254: v36,20.38 36,36 R24.1 | v42.38,12 v44.25,13.88
  Bottom 0.254: v36,20.38 38.88,17.5 39.62,17.5 IC10.16 39.75,17.38 41.38,17.38 41.38,14.5 40.75,13.88 38,13.88 38,12 38.62,11.38 41.75,11.38 v42.38,12 | v44.25,13.88 50.75,13.88 54.25,17.38 IC9.16
N$77  (via drill 0.61)
  Top 0.254: 49,35 50,36 R23.1 | 49,24.25 49,35 | 49,24.25 47.38,22.62 IC10.5 | v46.12,35.5 46.12,36.88 46,37 C4.2 | v48.62,35.25 48.88,35 49,35 | 49,24.25 49,19 58.62,19 61.96,22.34 IC9.5
  Bottom 0.254: v46.12,35.5 46.38,35.25 v48.62,35.25
N$78
  Top 0.813: C32.- 201,126.85 X7.6
N$79
  Top 0.813: C31.- 210.9,129.25 X7.8
N$80  (via drill 0.6 pad 0.25)
  other vias: 192.05,109.5
N$81  (via drill 0.6 pad 0.25)
  other vias: 187.45,109.4
N$82  (via drill 0.6 pad 0.25)
  other vias: 196.4,109.5
N$83  (via drill 0.6 pad 0.25)
  other vias: 192,116
N$84  (via drill 0.6 pad 0.25)
  other vias: 204.75,115.9
N$85  (via drill 0.6 pad 0.25)
  other vias: 214.9,115.85
N$86  (via drill 0.6 pad 0.25)
  other vias: 198.95,105.45
N$87  (via drill 0.6 pad 0.25)
  other vias: 188.1,105.1
N$88  (via drill 0.6)
  other vias: 213,110
N$89  (via drill 0.6)
  other vias: 212.15,96.35
N$90  (via drill 0.6)
  other vias: 202.1,96.4
N$91  (via drill 0.6 pad 2.18)
  other vias: 9.7,105.55
N$93  (via drill 1 pad 1.78)
  other vias: 9.41,99.06
N$94  (via drill 1 pad 1.78)
  other vias: 9.41,96.52
N$95  (via drill 1 pad 1.78)
  other vias: 9.41,93.98
N$96  (via drill 1 pad 1.78)
  other vias: 9.41,91.44
N$97  (via drill 1 pad 1.78)
  other vias: 9.41,88.9
N$98  (via drill 1 pad 1.78)
  other vias: 9.41,86.36
N$99  (via drill 1 pad 1.78)
  other vias: 9.41,83.82
N$100  (via drill 1 pad 1.78)
  other vias: 9.41,81.28
N$101  (via drill 1 pad 1.78)
  other vias: 9.41,78.74
N$102  (via drill 1 pad 1.78)
  other vias: 9.41,76.2
N$103  (via drill 1 pad 1.78)
  other vias: 6.87,76.2
N$104  (via drill 1 pad 1.78)
  other vias: 6.87,78.74
N$105  (via drill 1 pad 1.78)
  other vias: 6.87,81.28
N$106  (via drill 1 pad 1.78)
  other vias: 6.87,83.82
N$107  (via drill 1 pad 1.78)
  other vias: 6.87,86.36
N$108  (via drill 1 pad 1.78)
  other vias: 6.87,88.9
N$109  (via drill 1 pad 1.78)
  other vias: 6.87,91.44
N$110  (via drill 1 pad 1.78)
  other vias: 6.87,93.98
N$111  (via drill 1 pad 1.78)
  other vias: 6.87,96.52
N$112  (via drill 1 pad 1.78)
  other vias: 6.87,99.06
N$113  (via drill 1 pad 1.78)
  other vias: 4.33,99.06
N$114  (via drill 1 pad 1.78)
  other vias: 4.33,96.52
N$115  (via drill 1 pad 1.78)
  other vias: 4.33,93.98
N$116  (via drill 1 pad 1.78)
  other vias: 4.33,91.44
N$117  (via drill 1 pad 1.78)
  other vias: 4.33,88.9
N$118  (via drill 1 pad 1.78)
  other vias: 4.33,86.36
N$119  (via drill 1 pad 1.78)
  other vias: 4.33,83.82
N$120  (via drill 1 pad 1.78)
  other vias: 4.33,81.28
N$121  (via drill 1 pad 1.78)
  other vias: 4.33,78.74
N$122  (via drill 1 pad 1.78)
  other vias: 4.33,76.2
N$123  (via drill 1 pad 1.78)
  other vias: 9.51,71.7
N$124  (via drill 1 pad 1.78)
  other vias: 6.97,71.7
N$125  (via drill 1 pad 1.78)
  other vias: 4.43,71.7
N$126
  Top 0.406: T4.B 153.86,103.14 156.76,100.24 R46.1 156.76,93.76 155,92 155,90.3 R56.2
PBANK  (via drill 0.61)
  Top 0.254: v73.38,119.25 71.5,121.12 v71.5,122.25 71.5,126.42 CN1.13 | v58.48,122.17 58.48,117.03 57.45,116 57.45,113.2 56.5,112.25 56.5,65.88 56.88,65.5 56.88,59.75 55.5,58.38 v55.5,57.38 | v21.25,55.38 21.25,54.38 13,46.12 13,39 15.6,36.4 IC1.12
  Bottom 0.254: v21.25,55.38 23.07,57.2 55.33,57.2 v55.5,57.38 | v71.5,122.25 58.55,122.25 v58.48,122.17 | v73.38,119.25 95.12,119.25 95.5,118.88 105.5,118.88 105.5,110.12 IC4.9
R  (via drill 0.61)
  Top 0.254: v144.38,110.75 144.38,109.75 144.88,109.25 R43.2 | v109.88,96.75 106.62,93.5 106.62,86.12 104,83.5 104,74.12 v103.62,73.75 | v106.75,70.62 107.12,70.25 107.12,45.38 108.25,44.25 108.25,40.25 107.38,39.38 107.38,37.12 108.12,36.38 108.12,14.5 v107.75,14.12 | v103.2,14.12 102.88,14.12 101.26,15.74 IC11.11
  Bottom 0.254: v144.38,110.75 144,110.38 116.25,110.38 116.25,102.75 | IC21.11 118.12,102.88 116.38,102.88 116.25,102.75 | JP3.1 126,11.38 123.25,14.12 v107.75,14.12 v103.2,14.12 | 116.25,102.75 110.25,96.75 v109.88,96.75 | v106.75,70.62 v103.62,73.75
RES  (via drill 0.61)  (1 unrouted)
  Top 0.254: 8.25,28.88 IC1.6 | 15.75,28.88 IC1.9 | v26.12,29.5 27,30.38 27,69.9 31.3,69.9 32.25,70.85 32.25,79 31.15,80.1 27.9,80.1 26.55,81.45 26.55,101.15 27.8,102.4 28.8,102.4 30.25,103.85 30.25,125.12 31.62,126.5
  Top 0.813: 15.75,28.88 8.25,28.88
  Bottom 0.254: IC1.9 15.88,28.88 25.5,28.88 v26.12,29.5
SL  (via drill 0.6)
  Top 0.254: 150.12,78.12 C8.-
  Top 0.406: v148.05,130.8 156.38,130.8 X3.7 156.38,127.38 155,126 148,126 148,122 148.6,121.4 148.6,99.4 151,97 151,79 150.12,78.12
  Bottom 0.406: v148.05,130.8 133.8,130.8 132,129 118,129 X1.1
SOUND-IN  (via drill 0.61)
  Top 0.254: v49,112.88 49,124.25 46.75,126.5 CN1.33 | v90.12,105 91.75,103.38 91.75,97.75 v96,93.5 | 151.78,67.78 v152,68
  Top 0.406: R37.2 151.78,67.78 153.3,66.25 165,66.25 167.35,68.6 R29.2 | v139.62,73.62 140,74 140,79 133,86 124,86 122,88 122,92 120.25,93.75 v120,93.75
  Bottom 0.254: v49,112.88 55.75,106.12 89,106.12 v90.12,105 | v96,93.5 96.25,93.75 v120,93.75 | v139.62,73.62 145.25,68 v152,68
SR  (via drill 0.6, 0.61)  (1 unrouted)
  Top 0.254: 167.88,78.25 C7.-
  Top 0.406: v159.15,129.7 X3.6 | 167.88,78.25 167.82,78.3 v167.82,91.55
  Bottom 0.406: v167.82,91.55 171.6,97.88 171.6,121.62 164.12,121.62 162.4,123.35 162.4,127.4 162.38,127.42 X3.6 | 130.75,125.38 131.68,125.38 136.05,129.75 146.25,129.75 147,129 149.75,129 150.45,129.7 v159.15,129.7
SYNC  (via drill 0.61)
  Top 0.254: JP3.7 118.38,11.38 112.25,17.5 v112.25,22.75 | 77.12,26.62 IC11.43 79.71,26.74 80.25,26.2 80.25,25.07 v81.08,24.25 | v148.25,68.88 148.62,68.5 148.62,39.25 146.88,37.5 141.25,37.5 141.25,33.12 138.12,30 v138.12,28.25
  Top 0.406: v153,75.88 153,95 154.01,96.01 R46.2
  Bottom 0.254: v81.08,24.25 111.62,24.25 112.25,23.62 | v153,75.88 148.25,71.12 v148.25,68.88 | v138.12,28.25 136.5,26.62 115.25,26.62 112.25,23.62 | v112.25,22.75 112.25,23.62
TO  (via drill 0.61)
  Top 0.254: IC11.13 99.08,17.77 101.22,17.77 102.62,16.38 v102.62,16 | v192.18,17.3 192.18,19.85 v192.43,20.1
  Bottom 0.254: v102.62,16 122.88,16 123.75,15.12 180.62,15.12 181.75,16.25 191.12,16.25 v192.18,17.3 | IC12.21 226.5,54.5 213,41 195.25,41 194.8,40.55 194.8,22.48 v192.43,20.1

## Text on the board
tNames: 9 | 8 | 7 | 6 | 5V-0.5A | 5 | 4 | 3 | 2 | 1 | + | + | CARTRIDGE SLOT | Audio Out | CXA1645 / not R67 | + | + | CXA2075 / not R66 R71 C36 C34 C35 | + | + | k | k | e | e | b | b | b | b | CXA1645M | e | e | k | k | 1 | + | T1-T4 - KT503 | 2 | 3 | R | G | B | S | + | + | JP1 | 1-2 27C010 | 2-3 27C256/512 | ALF-02 | by Dmitry Pugachev and Sergey Bagan aka Prusak | IC11 - plastic/keramika / R23 - 33/0 om / C4 - 33/100 pF | + | + | JOY-1 | JOY-2 | + | 9 | 1 | 10 | 2
201bmp: G:/Platform/Ýëüô/alf0.bmp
